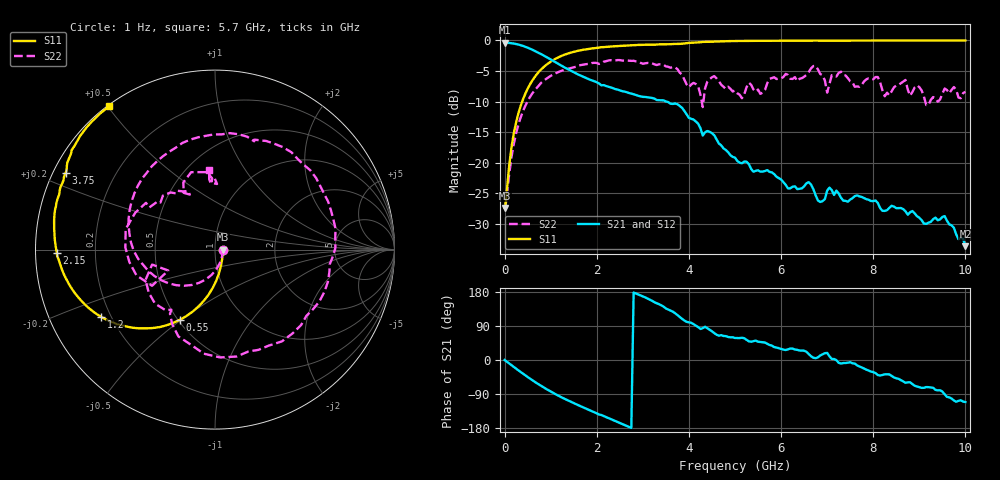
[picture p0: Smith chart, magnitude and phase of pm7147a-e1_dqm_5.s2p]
# GHz S DB R 50
! S-Parameters data
! Freq  dbS11  angS11  dbS21  angS21  dbS12  angS12  dbS22  angS22
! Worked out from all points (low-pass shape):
!   279 points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, 1 Hz to 10 GHz, reference 50 ohm
!   highest |S21| = -0.38 dB at 39.81 kHz (marker M1); lowest = -33.6 dB at 10 GHz (marker M2)
!   |S21| within 3 dB of the highest: start of sweep to 1.062 GHz
!   lowest |S11| = -27.4 dB at 39.81 kHz (marker M3), VSWR 1.09, Z = 54.4 - j0.00359 ohm
!   |S11| at or under -10 dB: start of sweep to 381.7 MHz
!   |S22| runs from -27.4 to -3.2 dB; largest |S21 - S12| = 0
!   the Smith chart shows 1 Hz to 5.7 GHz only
!   S11 on the Smith chart (normalised r, x): 1 Hz: 1.09, -0.00; 550 MHz: 0.51, -0.49; 1.2 GHz: 0.16, -0.27; 2.15 GHz: 0.06, -0.01; 3.75 GHz: 0.04, +0.24; 5.7 GHz: 0.00, +0.50
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1e-09  -27.41 -0.0  -0.38 -0.0  -0.38 -0.0  -27.41 -0.0
3.98107e-05  -27.41 -0.0  -0.38 -0.0  -0.38 -0.0  -27.41 -0.0
0.2  -15.17 -87.9  -0.51 -18.4  -0.51 -18.4  -16.90 -97.9
0.55  -7.20 -116.5  -1.35 -49.1  -1.35 -49.1  -9.26 -150.2
1.2  -2.65 -149.5  -3.97 -96.3  -3.97 -96.3  -5.07 140.5
1.7  -1.54 -167.0  -5.91 -124.7  -5.91 -124.7  -3.97 98.4
2.15  -1.10 -178.9  -7.31 -147.9  -7.31 -147.9  -3.49 64.6
2.8  -0.77 167.6  -8.80 178.0  -8.80 178.0  -3.33 10.1
3.35  -0.65 158.3  -9.78 147.4  -9.78 147.4  -3.90 -41.3
3.75  -0.58 152.7  -10.42 118.4  -10.42 118.4  -4.68 -96.2
4.2  -0.33 146.6  -13.61 87.0  -13.61 87.0  -7.48 -156.4
4.3  -0.24 145.2  -15.56 84.0  -15.56 84.0  -10.90 -155.9
4.5  -0.21 142.2  -15.17 75.8  -15.17 75.8  -6.03 178.6
4.65  -0.16 140.1  -16.86 64.2  -16.86 64.2  -6.66 145.9
5.05  -0.09 134.5  -19.71 58.0  -19.71 58.0  -8.65 118.7
5.7  -0.07 126.5  -21.21 42.9  -21.21 42.9  -7.00 94.2
6.7  -0.04 115.8  -24.33 6.0  -24.33 6.0  -4.19 30.4
6.95  -0.04 113.3  -25.95 18.0  -25.95 18.0  -6.53 2.5
8.35  -0.02 101.3  -27.37 -38.0  -27.37 -38.0  -8.97 -54.8
8.95  -0.02 96.8  -28.74 -69.8  -28.74 -69.8  -7.34 -99.2
9.15  -0.01 95.3  -29.99 -71.4  -29.99 -71.4  -10.57 -118.6
10  -0.01 89.6  -33.64 -111.1  -33.64 -111.1  -8.41 173.9
